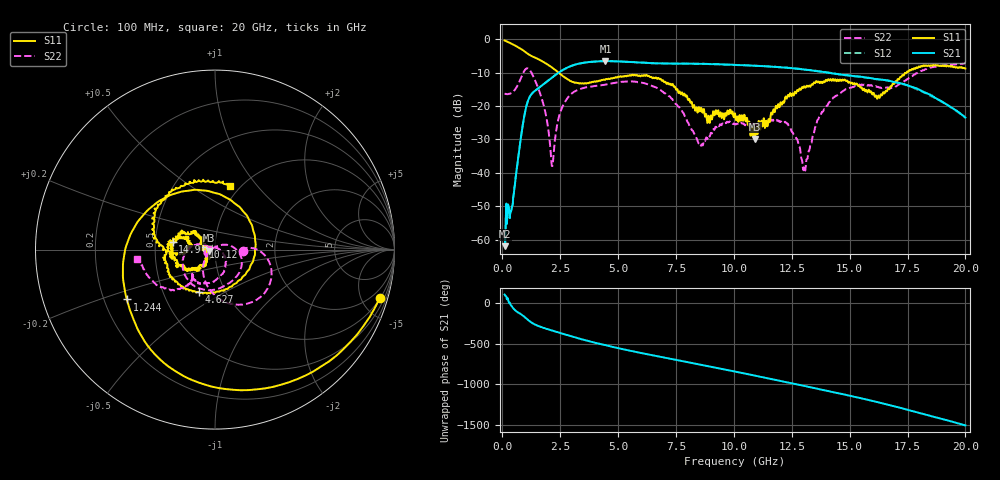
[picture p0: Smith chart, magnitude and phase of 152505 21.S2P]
!  2-Port S-parameters saved by WinCal
! VAR MeasName=S-Parameters (CALIBRATED_DATA) read from VNA (N5230C)
! VAR MeasDate=4/10/2015 9:30:21 AM
! VAR NAME=152505 21
! VAR FILENAME=152505 21.S2P
! VAR DATE=4/10/2015 9:30:21 AM
! VAR PHYS_PORTS=1,2
# Hz S DB R 50
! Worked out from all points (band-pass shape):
!   801 points, 100 MHz to 20 GHz, reference 50 ohm
!   highest |S21| = -6.57 dB at 4.453 GHz (marker M1); lowest = -61.9 dB at 124.9 MHz (marker M2)
!   |S21| within 3 dB of the highest: 2.528 GHz to 13.58 GHz (11.05 GHz wide, 137 % of centre)
!   lowest |S11| = -29.8 dB at 10.92 GHz (marker M3), VSWR 1.07, Z = 46.9 - j0.489 ohm
!   |S11| at or under -10 dB: 2.425 GHz to 17.46 GHz (15.03 GHz wide, 151 % of centre)
!   |S22| runs from -39.3 to -7.2 dB; largest |S21 - S12| = 0.0075
!   S11 on the Smith chart (normalised r, x): 100 MHz: 1.05, -6.79; 1.244 GHz: 0.30, -0.24; 4.627 GHz: 0.75, -0.38; 10.12 GHz: 0.88, +0.02; 14.9 GHz: 0.62, +0.05; 20 GHz: 0.90, +0.73
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1e8  -0.38 -16.4  -58.31 105.2  -57.87 110.2  -16.27 -2.2
1.24875e8  -0.46 -20.0  -61.92 94.0  -60.89 93.2  -16.33 -2.3
5.975e8  -2.07 -82.4  -40.36 -99.8  -40.30 -99.5  -14.59 3.2
1.24425e9  -4.97 -150.5  -16.59 122.9  -16.57 122.9  -9.81 -71.0
1.7915e9  -6.87 158.5  -13.42 52.9  -13.40 52.7  -19.88 -129.0
2.164625e9  -8.56 120.0  -11.36 19.7  -11.36 19.5  -37.95 110.1
2.612375e9  -11.05 67.1  -9.20 -18.9  -9.24 -19.0  -19.97 8.6
3.43325e9  -13.28 -35.2  -7.15 -87.0  -7.15 -86.8  -14.76 -40.5
4.453125e9  -12.10 -104.0  -6.57 -160.4  -6.56 -160.5  -13.60 -76.3
4.62725e9  -11.92 -110.5  -6.57 -172.1  -6.58 -172.0  -13.34 -82.3
6.741625e9  -11.58 170.4  -7.23 61.9  -7.20 61.5  -14.77 -166.0
8.5575e9  -21.41 138.6  -7.39 -39.8  -7.36 -39.8  -32.08 -171.5
1.005e10  -22.17 175.7  -7.68 -125.2  -7.70 -125.4  -25.48 -148.0
1.012462e10  -23.55 167.8  -7.70 -129.5  -7.72 -129.4  -25.29 -148.1
1.092062e10  -29.82 -170.7  -7.96 -175.5  -7.96 -175.3  -25.27 -149.1
1.228875e10  -17.77 -131.6  -8.53 103.5  -8.52 103.3  -25.22 -176.6
1.3035e10  -14.12 -144.3  -9.09 57.9  -9.03 57.4  -38.05 77.5
1.338325e10  -13.58 -153.2  -9.37 36.6  -9.30 36.5  -29.84 -14.4
1.490062e10  -12.42 170.3  -10.78 -56.7  -10.81 -57.9  -14.80 -94.7
1.669162e10  -14.93 -171.0  -12.42 -176.6  -12.47 -177.5  -14.51 -130.2
1.81095e10  -8.01 149.3  -15.52 76.4  -15.54 76.0  -9.52 -137.9
2e10  -8.77 76.8  -23.45 -70.3  -23.49 -69.5  -7.16 -173.1
